(* Data point pending state *)
TYPE ST_IEC870_5_101SPendingState :
STRUCT
	bSpont	: BOOL;(* TRUE => Send/received spontaneous data *)
	bCyclic	: BOOL;(* TRUE => Send cylclic data *)
	bGenin 	: BOOL;(* TRUE => Send general interrogation data *)
	bCoro	: BOOL;(* TRUE => Send counter interrogation data *)
END_STRUCT
END_TYPE
